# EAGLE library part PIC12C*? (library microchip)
MICROCONTROLLER
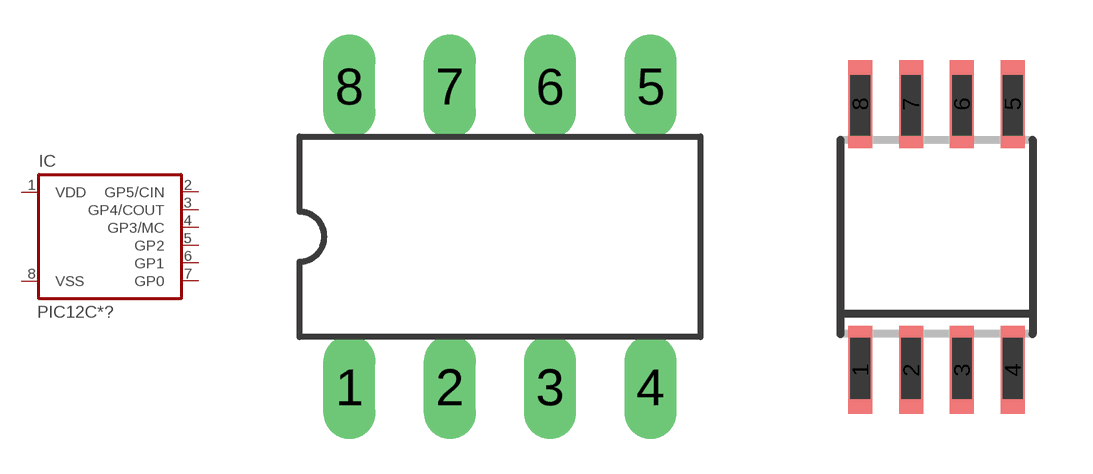
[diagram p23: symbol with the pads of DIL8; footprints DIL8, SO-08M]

Designator prefix IC

## PIC12C508P (MF: MICROCHIP; MPN: PIC12C508A-04I/P; OC_FARNELL: 9758763; OC_NEWARK: 12C1849), PIC12C509P (MF: MICROCHIP; MPN: PIC12C509-04/P; OC_FARNELL: 9758810; OC_NEWARK: 54K2820), PIC12C671P (MF: MICROCHIP; MPN: PIC12C671-10/P; OC_FARNELL: 9758860; OC_NEWARK: 23C2974), PIC12C672P (MF: MICROCHIP; MPN: PIC12C672-04/P; OC_FARNELL: 9758887; OC_NEWARK: 59K0241)  [DIL8]
1  VDD  pwr
2  GP5/CIN
3  GP4/COUT
4  GP3/MC  in
5  GP2
6  GP1
7  GP0
8  VSS  pwr

## PIC12C508JN (MF: MICROCHIP; MPN: PIC12C508-04/P; OC_FARNELL: 9758771; OC_NEWARK: 60K6710), PIC12C509JN (MF: MICROCHIP; MPN: PIC12C509A-04I/P; OC_FARNELL: 9758828; OC_NEWARK: 23C2958), PIC12C671JN (MPN: PIC12C671-10I/P; OC_FARNELL: 1084238; OC_NEWARK: 34M7956), PIC12C672JN (MF: MICROCHIP; MPN: PIC12C672-04/P; OC_FARNELL: 9758887; OC_NEWARK: 59K0241)  [DIL8]
Pads as for DIL8

## PIC12C508SM (MF: MICROCHIP; MPN: PIC12C508-04I/SM; OC_FARNELL: 1196846; OC_NEWARK: 96K3762), PIC12C509SM (MF: MICROCHIP; MPN: PIC12C509A-04I/SM; OC_FARNELL: 9758844; OC_NEWARK: 65K1035), PIC12C671SM (MPN: PIC12C671-10I/SM; OC_FARNELL: 1196776; OC_NEWARK: 24M5845), PIC12C672SM (MF: MICROCHIP; MPN: PIC12C672-04/SM; OC_FARNELL: 1137297; OC_NEWARK: 72K7294)  [SO-08M]
Pads as for DIL8

## Footprint DIL8 (pad centres in mm)
Dual In Line package type P
drill 0.813 long: 1 -3.81,-3.81; 2 -1.27,-3.81; 3 1.27,-3.81; 4 3.81,-3.81; 5 3.81,3.81; 6 1.27,3.81; 7 -1.27,3.81; 8 -3.81,3.81

## Footprint SO-08M (pad centres in mm)
Small Outline Medium Plastic Gull Wing 207-mil body, package type SM
smd 0.6 x 2.2: 1 -1.905,-3.33; 2 -0.635,-3.33; 3 0.635,-3.33; 4 1.905,-3.33; 5 1.905,3.33; 6 0.635,3.33; 7 -0.635,3.33; 8 -1.905,3.33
